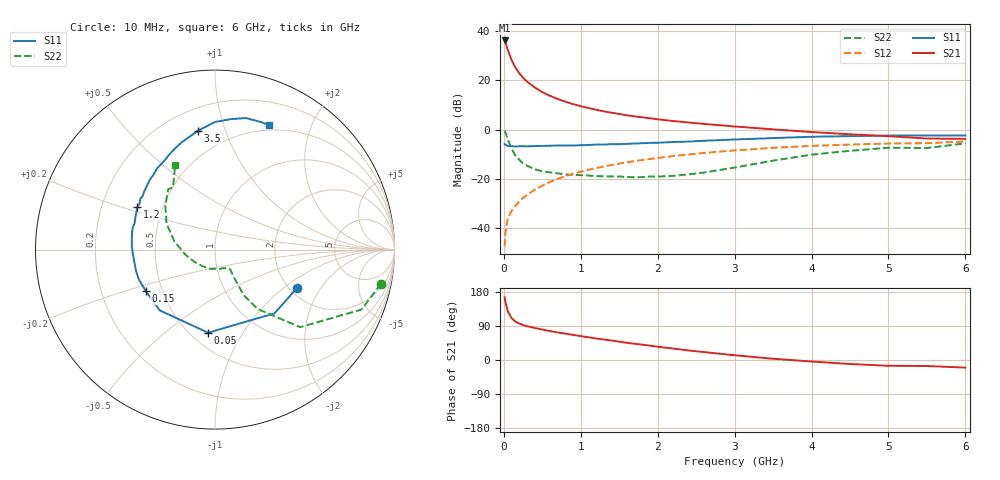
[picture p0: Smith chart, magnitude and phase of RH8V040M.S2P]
! SIEMENS Small Signal Semiconductors
! BFR106
! Si NPN RF Bipolar Junction Transistor in SOT23
! VCE = 8 V  IC = 40 mA
! Common Emitter S-Parameters:  August  1996
# GHz  S  MA  R  50
!  f  S11  S21  S12  S22
! GHz  MAG  ANG  MAG  ANG  MAG  ANG  MAG  ANG
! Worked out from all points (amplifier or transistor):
!   36 points, 10 MHz to 6 GHz, reference 50 ohm
!   highest |S21| = 36.3 dB at 10 MHz (marker M1)
!   |S21| within 3 dB of that: start of sweep to 43.49 MHz
!   unconditionally stable (mu >= 1): 284.1 MHz to 2.196 GHz
!   at 250 MHz: K = 0.97, MSG = 24.5 dB, |S12| = -27.9 dB
!   at 1.4 GHz: K = 1.06, MAG = 9.2 dB, |S12| = -14.5 dB
!   at 6 GHz: K = 0.98, MSG = 0.5 dB, |S12| = -4.9 dB
!   S11 on the Smith chart (normalised r, x): 10 MHz: 2.21, -1.25; 50 MHz: 0.61, -0.72; 150 MHz: 0.40, -0.23; 1.2 GHz: 0.36, +0.22; 3.5 GHz: 0.34, +0.81; 6 GHz: 0.44, +1.43
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0.01  0.5056 -24.7  65.18 165.4  0.0042 83.3  0.9439 -11.6
0.02  0.4859 -47.0  60.01 153.9  0.0077 74.8  0.8827 -22.2
0.05  0.4646 -94.8  42.9 129.2  0.0152 60.3  0.6422 -42.3
0.1  0.4578 -132.3  26.25 110.8  0.022 60.5  0.4065 -54.4
0.15  0.4499 -149.3  18.34 101.5  0.0278 61.4  0.2977 -57.9
0.2  0.4559 -158.8  14.09 96.4  0.0339 64.5  0.2418 -56.9
0.25  0.4554 -165.5  11.36 92.3  0.0404 65.6  0.2033 -56.2
0.3  0.4543 -169.8  9.514 89.4  0.0463 68.0  0.184 -55.7
0.4  0.4585 -177.4  7.219 84.7  0.0592 69.7  0.1554 -53.8
0.5  0.4638 177.7  5.79 80.3  0.0721 70.2  0.1408 -52.3
0.6  0.4673 172.4  4.855 76.3  0.0856 70.4  0.134 -53.3
0.7  0.4713 168.7  4.195 72.7  0.0988 69.9  0.1277 -54.9
0.9  0.4715 161.5  3.294 66.2  0.1253 68.4  0.1184 -57.4
1.1  0.485 154.5  2.74 59.9  0.1509 66.3  0.1153 -64.9
1.2  0.4933 151.4  2.528 56.8  0.1637 65.3  0.1123 -68.5
1.6  0.5106 140.6  1.948 45.5  0.2142 60.2  0.108 -86.6
2.2  0.5563 125.4  1.489 30.2  0.2869 52.2  0.1133 -122.2
2.8  0.6072 111.3  1.225 16.7  0.3533 43.5  0.1495 -161.2
3.5  0.6687 98.2  1.007 3.3  0.4238 33.3  0.232 168.3
4.5  0.7324 83.0  0.8 -10.5  0.4924 18.5  0.3682 138.7
5.5  0.7552 70.4  0.655 -15.9  0.5266 8.4  0.4192 123.9
6  0.7567 66.5  0.645 -20.1  0.5692 1.1  0.5229 115.1
